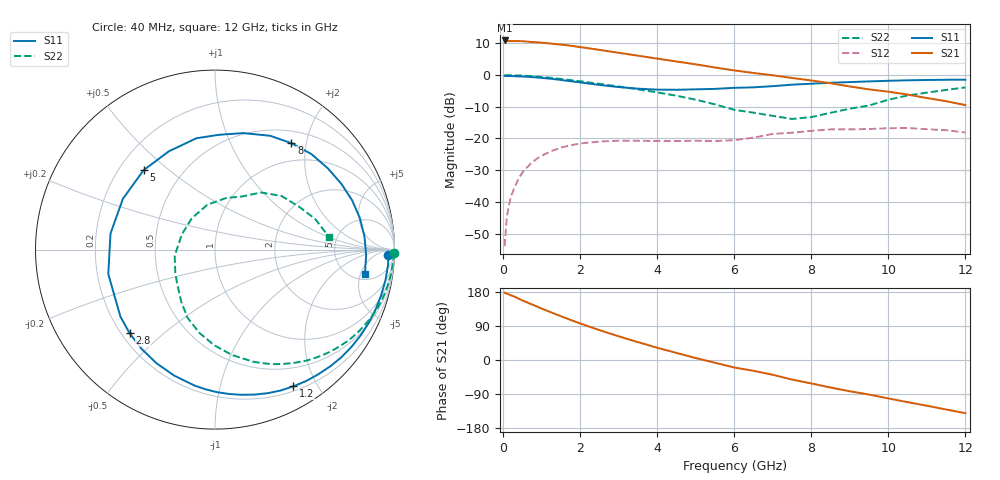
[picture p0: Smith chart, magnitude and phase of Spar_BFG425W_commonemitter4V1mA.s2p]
! Filename: 41bfg425.001
! BFG425W Field C1
! V1=7.837E-001V,V2=4.000E+000V, I1=8.591E-006A, I2=1.000E-003A
# GHz  S  MA  R 50
!  S11  S21  S12  S22
!Freq(GHz)  Mag  Ang  Mag  Ang  Mag  Ang  Mag  Ang
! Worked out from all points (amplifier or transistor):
!   44 points, 40 MHz to 12 GHz, reference 50 ohm
!   highest |S21| = 10.9 dB at 40 MHz (marker M1)
!   |S21| within 3 dB of that: start of sweep to 2.517 GHz
!   unconditionally stable (mu >= 1): 3.429 GHz to end of sweep
!   at 700 MHz: K = 0.13, MSG = 19.3 dB, |S12| = -28.2 dB
!   at 2.4 GHz: K = 0.55, MSG = 14.6 dB, |S12| = -21.1 dB
!   at 12 GHz: K = 2.23, MAG = -1.9 dB, |S12| = -18.1 dB
!   S11 on the Smith chart (normalised r, x): 40 MHz: 35, -29; 1.2 GHz: 0.25, -1.70; 2.8 GHz: 0.23, -0.39; 5 GHz: 0.30, +0.41; 8 GHz: 0.69, +1.74; 12 GHz: 6.13, -5.95
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0.04  0.967 -1.6  3.513 177.6  0.002 70.9  0.995 -1.1
0.1  0.968 -5.1  3.444 175.3  0.006 83.8  0.995 -2.8
0.2  0.965 -10.2  3.433 170.8  0.012 80.9  0.992 -5.7
0.4  0.955 -20.3  3.432 162.0  0.023 74.6  0.984 -11.3
0.6  0.942 -30.4  3.38 152.9  0.034 68.2  0.971 -16.8
0.8  0.925 -40.4  3.306 144.5  0.044 61.3  0.953 -22.2
1.2  0.878 -60.2  3.156 127.6  0.061 48.6  0.908 -32.5
1.5  0.837 -74.8  3.023 115.6  0.072 39.6  0.868 -39.8
1.7  0.808 -84.5  2.932 107.8  0.077 34.1  0.84 -44.4
2.2  0.738 -107.9  2.654 89.4  0.086 21.5  0.769 -55.2
2.8  0.666 -135.6  2.342 69.0  0.091 9.3  0.686 -67.3
3.5  0.61 -167.1  2.022 47.2  0.092 -1.2  0.595 -80.8
4  0.589 171.3  1.818 32.4  0.091 -6.7  0.533 -90.5
4.5  0.586 151.1  1.638 18.7  0.091 -10.4  0.472 -100.6
5  0.595 132.0  1.475 5.2  0.092 -14.9  0.409 -112.1
6  0.629 99.5  1.183 -19.8  0.094 -21.7  0.283 -138.2
6.5  0.64 88.0  1.079 -28.5  0.103 -15.2  0.255 -150.3
7.5  0.705 64.0  0.899 -51.6  0.123 -30.8  0.203 155.1
8  0.73 54.3  0.821 -61.8  0.132 -36.6  0.217 126.7
8.5  0.756 44.8  0.744 -72.6  0.139 -45.5  0.254 99.5
10.5  0.826 12.3  0.492 -111.3  0.146 -80.1  0.476 38.9
12  0.846 -9.4  0.336 -140.4  0.124 -112.5  0.638 6.5
